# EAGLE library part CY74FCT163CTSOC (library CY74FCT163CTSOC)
Counter ICs Synch 4B Bin Counter Source: Datasheet
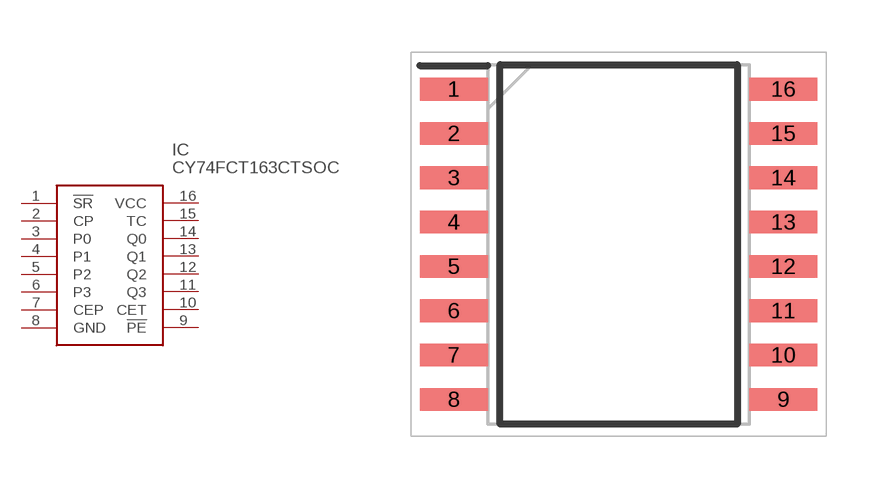
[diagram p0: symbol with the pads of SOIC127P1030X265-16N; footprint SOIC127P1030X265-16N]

Designator prefix IC

## CY74FCT163CTSOC (Description: Counter ICs Synch 4B Bin Counter; Height: 2.65mm; Manufacturer_Name: Texas Instruments; Manufacturer_Part_Number: CY74FCT163CTSOC; Mouser_Part_Number: 595-CY74FCT163CTSOC; Mouser_Price-Stock: https://www.mouser.com/Search/Refine.aspx?Keyword=595-CY74FCT163CTSOC)  [SOIC127P1030X265-16N]
1  !SR
2  CP
3  P0
4  P1
5  P2
6  P3
7  CEP
8  GND
9  !PE
10  CET
11  Q3
12  Q2
13  Q1
14  Q0
15  TC
16  VCC

## Footprint SOIC127P1030X265-16N (pad centres in mm)
DW0016A_1
smd 1.95 x 0.65: 1 -4.725,4.445; 2 -4.725,3.175; 3 -4.725,1.905; 4 -4.725,0.635; 5 -4.725,-0.635; 6 -4.725,-1.905; 7 -4.725,-3.175; 8 -4.725,-4.445; 9 4.725,-4.445; 10 4.725,-3.175; 11 4.725,-1.905; 12 4.725,-0.635; 13 4.725,0.635; 14 4.725,1.905; 15 4.725,3.175; 16 4.725,4.445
